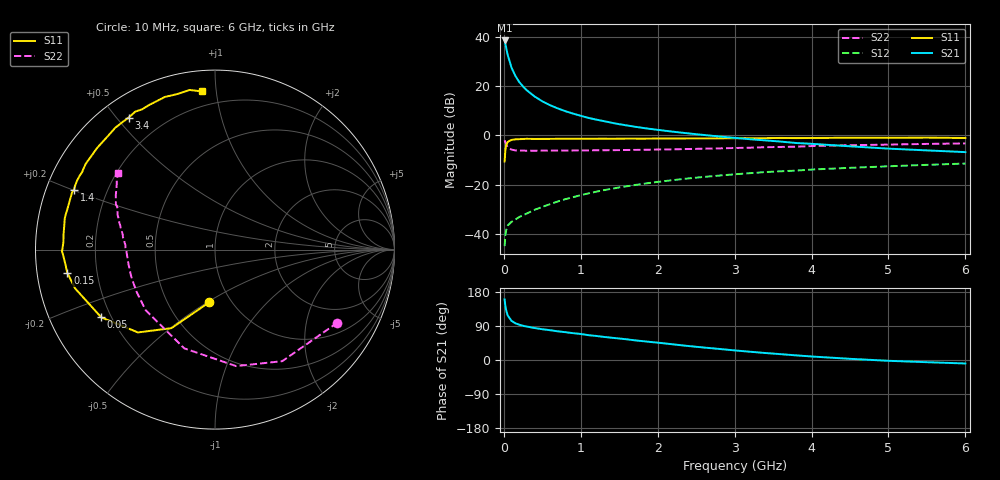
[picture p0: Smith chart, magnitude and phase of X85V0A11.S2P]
! SIEMENS Small Signal Semiconductors
! BFP136W
! Si NPN RF Bipolar Junction Transistor in SOT343
! VCE = 5 V  IC = 110 mA
! Common Emitter S-Parameters:  September  1994
# GHz  S  MA  R  50
!  f  S11  S21  S12  S22
! GHz  MAG  ANG  MAG  ANG  MAG  ANG  MAG  ANG
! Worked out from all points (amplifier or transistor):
!   40 points, 10 MHz to 6 GHz, reference 50 ohm
!   highest |S21| = 38.6 dB at 10 MHz (marker M1)
!   |S21| within 3 dB of that: start of sweep to 30.77 MHz
!   unconditionally stable (mu >= 1): 512 MHz to 2.964 GHz
!   at 200 MHz: K = 0.69, MSG = 27.4 dB, |S12| = -33.2 dB
!   at 1.5 GHz: K = 1.10, MAG = 11.0 dB, |S12| = -21.1 dB
!   at 6 GHz: K = 0.97, MSG = 2.3 dB, |S12| = -11.4 dB
!   S11 on the Smith chart (normalised r, x): 10 MHz: 0.79, -0.51; 50 MHz: 0.16, -0.27; 150 MHz: 0.09, -0.08; 1.4 GHz: 0.08, +0.20; 3.4 GHz: 0.08, +0.54; 6 GHz: 0.11, +0.91
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0.01  0.2955 -96.3  85 159.8  0.0056 67.6  0.7945 -30.8
0.02  0.5003 -119.0  72.61 143.2  0.0094 55.7  0.7259 -58.9
0.03  0.6301 -132.9  60.98 131.5  0.0117 49.1  0.6598 -79.7
0.05  0.7375 -149.2  43.26 117.5  0.0147 38.4  0.5762 -107.3
0.1  0.8089 -164.5  23.82 103.2  0.0175 36.2  0.5132 -138.8
0.15  0.8327 -171.0  16.2 96.9  0.0195 40.1  0.496 -151.8
0.2  0.8376 -174.4  12.17 93.1  0.0219 42.1  0.4909 -158.8
0.25  0.8449 -177.3  9.809 90.3  0.0238 44.9  0.4899 -163.3
0.3  0.8522 -179.3  8.201 88.1  0.0259 48.1  0.488 -166.3
0.4  0.8457 177.2  6.176 84.4  0.0307 51.3  0.4889 -170.4
0.5  0.8479 174.5  4.925 81.2  0.0352 54.8  0.4894 -173.1
0.6  0.8489 172.5  4.107 78.7  0.04 57.2  0.49 -174.9
0.7  0.852 169.9  3.541 75.7  0.0453 59.1  0.4911 -176.3
0.9  0.8542 166.5  2.772 70.8  0.0555 60.4  0.4933 -178.9
1.1  0.8536 161.9  2.266 65.5  0.0662 61.0  0.4966 179.5
1.4  0.8533 156.9  1.808 58.8  0.0821 60.5  0.5002 177.0
2.2  0.864 143.1  1.187 41.3  0.1233 55.1  0.5203 170.9
3.2  0.8777 126.1  0.835 21.8  0.1706 45.7  0.5623 162.3
3.4  0.8788 123.2  0.791 18.4  0.1796 43.5  0.5751 160.6
4.5  0.895 108.2  0.6 3.1  0.2192 33.4  0.6313 151.1
5.5  0.9005 99.0  0.495 -5.8  0.2519 25.6  0.6712 144.6
6  0.8842 94.7  0.457 -9.2  0.2679 21.3  0.6865 141.7
